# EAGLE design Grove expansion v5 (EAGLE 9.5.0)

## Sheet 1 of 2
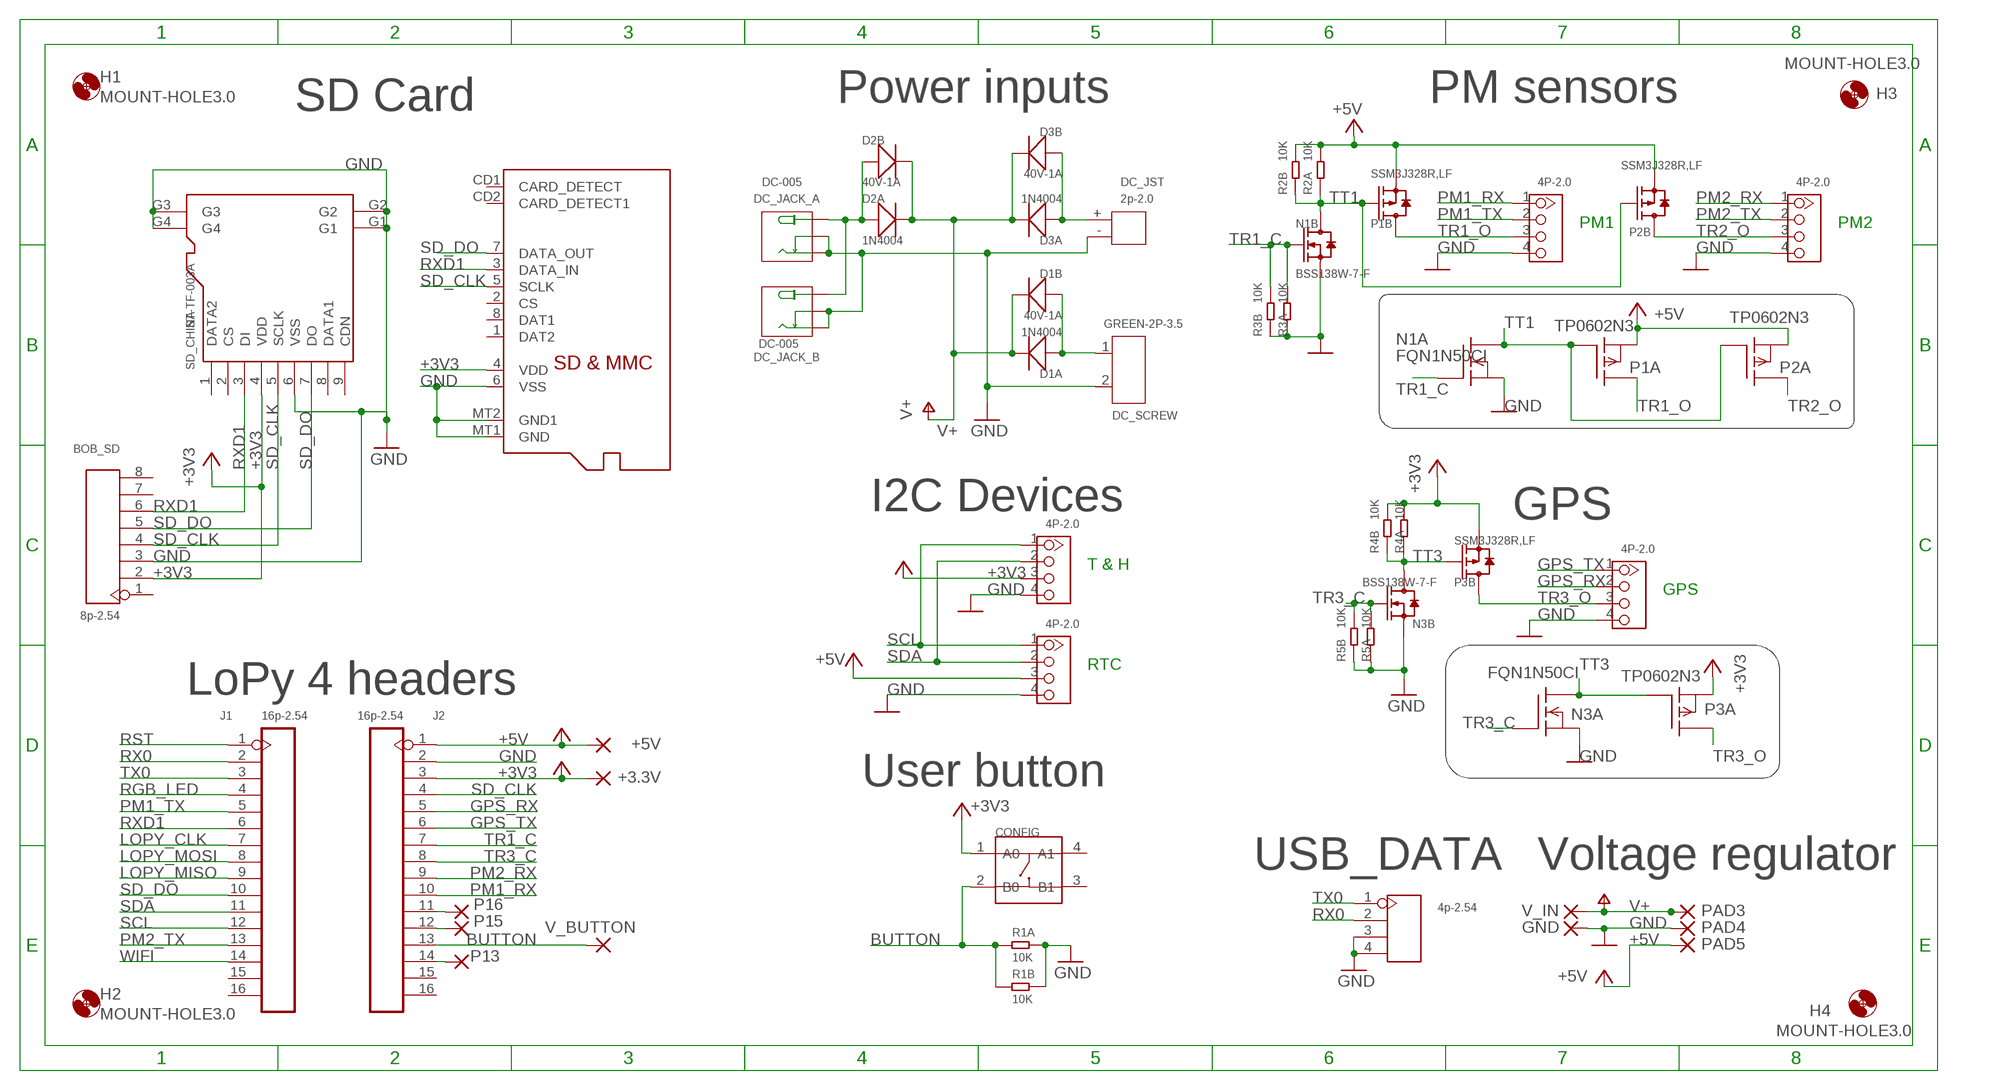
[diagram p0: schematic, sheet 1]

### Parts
+3.3V  3.3V  2,15/1,0  [2,15/1,0]
+5V  5V  2,15/1,0  [2,15/1,0]
BOB_SD  8p-2.54  DIP-BLACK-FEMALE-HEADER-VERT(8P-2.54)  [H8-2.54]
CONFIG  DIP-SWITCH-TACTILE-SPST-NO/TS-1109(4P-D6.0MM)'TS-1109'  [SW4-6.0X6.0X5.0MM]
D1A  1N4004  DIP-DIODE-400V-1A(DO-41)  [DO-41]
D1B  40V-1A  SMD-DIODE-SCHOTTKY-40V-1A(DO-214AC)  [DO-214AC]
D2A  1N4004  DIP-DIODE-400V-1A(DO-41)  [DO-41]
D2B  40V-1A  SMD-DIODE-SCHOTTKY-40V-1A(DO-214AC)  [DO-214AC]
D3A  1N4004  DIP-DIODE-400V-1A(DO-41)  [DO-41]
D3B  40V-1A  SMD-DIODE-SCHOTTKY-40V-1A(DO-214AC)  [DO-214AC]
DC_JACK_A  DC-005  CONN-POWER-JACK-2.1MM(DC-005)  [DCJ3P-14.2X11.0X9.0MM]
DC_JACK_B  DC-005  CONN-POWER-JACK-2.1MM(DC-005)  [DCJ3P-14.2X11.0X9.0MM]
DC_JST  2p-2.0  DIP-JST-2P-2.0  [H2-2.0-6X4.5MM]
DC_SCREW  GREEN-2P-3.5  SCREW-TERMINAL-GREEN(2P-3.5)  [H2-3.5-7.0X7.0MM]
GND  0V  2,15/1,0  [2,15/1,0]
GPS-(DIG)  4P-2.0  GROVE-CONNECTOR-DIP(4P-2.0)  [HW4-2.0]
H1  MOUNT-HOLE3.0  [3,0]
H2  MOUNT-HOLE3.0  [3,0]
H3  MOUNT-HOLE3.0  [3,0]
H4  MOUNT-HOLE3.0  [3,0]
J1  16p-2.54  DIP-BLACK-MALE-HEADER-VERT(16P-2.54)  [H16-2.54]
J2  16p-2.54  DIP-BLACK-MALE-HEADER-VERT(16P-2.54)  [H16-2.54]
N1A  FQN1N50CI  [TO92-INLINE]
N1B  BSS138W-7-F  SMD-MOSFET-N-CH-50V-200MA-BSS138W-7-F(SOT-23)  [SOT-23]
N3A  FQN1N50CI  [TO92-INLINE]
N3B  BSS138W-7-F  SMD-MOSFET-N-CH-50V-200MA-BSS138W-7-F(SOT-23)  [SOT-23]
P1A  TP0602N3  [TO-92]
P1B  SSM3J328R,LF  SMD-MOSFET-P-CH-20V-6A-SSM3J328R(SOT-23)  [SOT-23]
P2A  TP0602N3  [TO-92]
P2B  SSM3J328R,LF  SMD-MOSFET-P-CH-20V-6A-SSM3J328R(SOT-23)  [SOT-23]
P3A  TP0602N3  [TO-92]
P3B  SSM3J328R,LF  SMD-MOSFET-P-CH-20V-6A-SSM3J328R(SOT-23)  [SOT-23]
P13  2,15/1,0  [2,15/1,0]
P15  2,15/1,0  [2,15/1,0]
P16  2,15/1,0  [2,15/1,0]
PAD3  12V  1,6/0,8  [1,6/0,8]
PAD4  0V  1,6/0,8  [1,6/0,8]
PAD5  5V  1,6/0,8  [1,6/0,8]
PM1-(UART)  4P-2.0  GROVE-CONNECTOR-DIP(4P-2.0)  [HW4-2.0]
PM2-(UART)  4P-2.0  GROVE-CONNECTOR-DIP(4P-2.0)  [HW4-2.0]
R1A  10K  DIP-RES-10K-5%-1/4W(PR-D2.3XL6.5MM)  [PR-D2.3XL6.5MM]
R1B  10K  SMD-RES-10K-1%-1/10W(0603)  [R0603]
R2A  10K  DIP-RES-10K-5%-1/4W(PR-D2.3XL6.5MM)  [PR-D2.3XL6.5MM]
R2B  10K  SMD-RES-10K-1%-1/10W(0603)  [R0603]
R3A  10K  DIP-RES-10K-5%-1/4W(PR-D2.3XL6.5MM)  [PR-D2.3XL6.5MM]
R3B  10K  SMD-RES-10K-1%-1/10W(0603)  [R0603]
R4A  10K  DIP-RES-10K-5%-1/4W(PR-D2.3XL6.5MM)  [PR-D2.3XL6.5MM]
R4B  10K  SMD-RES-10K-1%-1/10W(0603)  [R0603]
R5A  10K  DIP-RES-10K-5%-1/4W(PR-D2.3XL6.5MM)  [PR-D2.3XL6.5MM]
R5B  10K  SMD-RES-10K-1%-1/10W(0603)  [R0603]
RTC-(I2C)  4P-2.0  GROVE-CONNECTOR-DIP(4P-2.0)  [HW4-2.0]
SD_CHINA  ST-TF-003A  MICRO-SD-CARD-SOCKET-9P(ST-TF-003A)  [MICRO-SD9+4P-SMD-16.1X14.5X1.85MM]
SD_UK  MICROSD  [MICROSD]
TH-(I2C)  4P-2.0  GROVE-CONNECTOR-DIP(4P-2.0)  [HW4-2.0]
USB_DATA  4p-2.54  DIP-BLACK-FEMALE-HEADER-VERT(4P-2.54)  [H4-2.54]
V_BUTTON  3.3V  2,15/1,0  [2,15/1,0]
V_IN  12V  2,15/1,0  [2,15/1,0]

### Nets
+3V3: +3.3V.1(P) BOB_SD.2 CONFIG.1(A0) J2.3 P3A.1(S) P3B.2(S) R4A.2 R4B.2 SD_CHINA.4(VDD) SD_UK.4(VDD) TH-(I2C).3
+5V: +5V.1(P) J2.1 P1A.1(S) P1B.2(S) P2A.1(S) P2B.2(S) PAD5.1(P) R2A.2 R2B.2 RTC-(I2C).3
BUTTON: CONFIG.2(B0) J2.13 R1A.1 R1B.1 V_BUTTON.1(P)
GND: BOB_SD.3 DC_JACK_A.-1(-) DC_JACK_A.-2(CDN) DC_JACK_B.-1(-) DC_JACK_B.-2(CDN) DC_JST.- DC_SCREW.2 GND.1(P) GPS-(DIG).4 J2.2 N1A.3(S) N1B.2(S) N3A.3(S) N3B.2(S) PAD4.1(P) PM1-(UART).4 PM2-(UART).4 R1A.2 R1B.2 R3A.1 R3B.1 R5A.1 R5B.1 RTC-(I2C).4 SD_CHINA.6(VSS) SD_CHINA.G1 SD_CHINA.G2 SD_CHINA.G3 SD_CHINA.G4 SD_UK.6(VSS) SD_UK.MT1(GND) SD_UK.MT2(GND1) TH-(I2C).4 USB_DATA.3 USB_DATA.4
GPS_RX: GPS-(DIG).2 J2.5
GPS_TX: GPS-(DIG).1 J2.6
JACK_V+: D2A.1(+) D2B.1(+) DC_JACK_A.+ DC_JACK_B.+
JST_V+: D3A.1(+) D3B.1(+) DC_JST.+
LOPY_CLK: J1.7
LOPY_MISO: J1.9
LOPY_MOSI: J1.8
P13: J2.14 P13.1(P)
P15: J2.12 P15.1(P)
P16: J2.11 P16.1(P)
PM1_RX: J2.10 PM1-(UART).1
PM1_TX: J1.5 PM1-(UART).2
PM2_RX: J2.9 PM2-(UART).1
PM2_TX: J1.13 PM2-(UART).2
RGB_LED: J1.4
RST: J1.1
RX0: J1.2 USB_DATA.2
RXD1: BOB_SD.6 J1.6 SD_CHINA.3(DI) SD_UK.3(DATA_IN)
SCL: J1.12 RTC-(I2C).1 TH-(I2C).1
SCREW_V+: D1A.1(+) D1B.1(+) DC_SCREW.1
SD_CLK: BOB_SD.4 J2.4 SD_CHINA.5(SCLK) SD_UK.5(SCLK)
SD_DO: BOB_SD.5 J1.10 SD_CHINA.7(DO) SD_UK.7(DATA_OUT)
SDA: J1.11 RTC-(I2C).2 TH-(I2C).2
TR1_C: J2.7 N1A.2(G) N1B.1(G) R3A.2 R3B.2
TR1_O: P1A.3(D) P1B.3(D) PM1-(UART).3
TR2_O: P2A.3(D) P2B.3(D) PM2-(UART).3
TR3_C: J2.8 N3A.2(G) N3B.1(G) R5A.2 R5B.2
TR3_O: GPS-(DIG).3 P3A.3(D) P3B.3(D)
TT1: N1A.1(D) N1B.3(D) P1A.2(G) P1B.1(G) P2A.2(G) P2B.1(G) R2A.1 R2B.1
TT3: N3A.1(D) N3B.3(D) P3A.2(G) P3B.1(G) R4A.1 R4B.1
TX0: J1.3 USB_DATA.1
V+: D1A.2(-) D1B.2(-) D2A.2(-) D2B.2(-) D3A.2(-) D3B.2(-) PAD3.1(P) V_IN.1(P)
WIFI: J1.14
Unconnected: BOB_SD.1 BOB_SD.7 BOB_SD.8 CONFIG.3(B1) CONFIG.4(A1) J1.15 J1.16 J2.15 J2.16 SD_CHINA.1(DATA2) SD_CHINA.2(CS) SD_CHINA.8(DATA1) SD_CHINA.9(CDN) SD_UK.1(DAT2) SD_UK.2(CS) SD_UK.8(DAT1) SD_UK.CD1(CARD_DETECT) SD_UK.CD2(CARD_DETECT1)

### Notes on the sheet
- SD Card | Power inputs | PM sensors
- PM1 | PM2
- I2C Devices | GPS
- T & H
- GPS
- RTC
- LoPy 4 headers
- User button
- Voltage regulator

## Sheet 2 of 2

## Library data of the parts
+3.3V +5V GND P13 P15 P16 V_BUTTON V_IN = wirepad:2,15/1,0: THROUGH-HOLE PAD
BOB_SD = OPL_Connector:DIP-BLACK-FEMALE-HEADER-VERT(8P-2.54): 320030061; MPN: F185-1108A1BSYC1
CONFIG = OPL_Switch:DIP-SWITCH-TACTILE-SPST-NO/TS-1109(4P-D6.0MM): 311020024
D1A D2A D3A = OPL_Discrete_Semiconductor:DIP-DIODE-400V-1A(DO-41): 304010008; MPN: 1N4004
D1B D2B D3B = OPL_Discrete_Semiconductor:SMD-DIODE-SCHOTTKY-40V-1A(DO-214AC): 304020027; MPN: 1N5819
DC_JACK_A DC_JACK_B = OPL_Connector:CONN-POWER-JACK-2.1MM(DC-005): 320120003; MPN: DC-005
DC_JST = OPL_Connector:DIP-JST-2P-2.0: 320110049
DC_SCREW = OPL_Connector:SCREW-TERMINAL-GREEN(2P-3.5): 320110028
GPS-(DIG) PM1-(UART) PM2-(UART) RTC-(I2C) TH-(I2C) = OPL_Connector:GROVE-CONNECTOR-DIP(4P-2.0): 320110033
H1-H4 = holes:MOUNT-HOLE: MOUNTING HOLE with drill center marker
J1 J2 = OPL_Connector:DIP-BLACK-MALE-HEADER-VERT(16P-2.54): 320020034; MPN: P125-1116A0BS116AX
N1A N3A = adafruit:FQN1N50C: N-Channel Enhancement MOSFET 500V, 0.4A, 6.0 Ohm
N1B N3B = OPL_Discrete_Semiconductor:SMD-MOSFET-N-CH-50V-200MA-BSS138W-7-F(SOT-23): 305030000; MPN: BSS138W-7-F
P1A P2A P3A = transistor-fet:TP0602N3: P-Channel Enhancement MOSFET -20V; -2A; 2,0Ohm
P1B P2B P3B = OPL_Discrete_Semiconductor:SMD-MOSFET-P-CH-20V-6A-SSM3J328R(SOT-23): 305030075; MPN: SSM3J328R,LF
PAD3-PAD5 = wirepad:1,6/0,8: THROUGH-HOLE PAD
R1A R2A R3A R4A R5A = OPL_Resistor:DIP-RES-10K-5%-1/4W(PR-D2.3XL6.5MM): 301020001; MPN: FHCFR-1/4W-103J
R1B R2B R3B R4B R5B = OPL_Resistor:SMD-RES-10K-1%-1/10W(0603): 301011970; MPN: RC0603FR-0710KL
SD_CHINA = OPL_Connector:MICRO-SD-CARD-SOCKET-9P(ST-TF-003A): 320090000; MPN: ST-TF-003A
SD_UK = adafruit:MICROSD: Micro-SD / Transflash card holder with SPI pinout For the 3M # 2908-05WB-MG and/or 4UCON #19656 push-push type
USB_DATA = OPL_Connector:DIP-BLACK-FEMALE-HEADER-VERT(4P-2.54): 320030017; MPN: F185-1104A1BSYA1

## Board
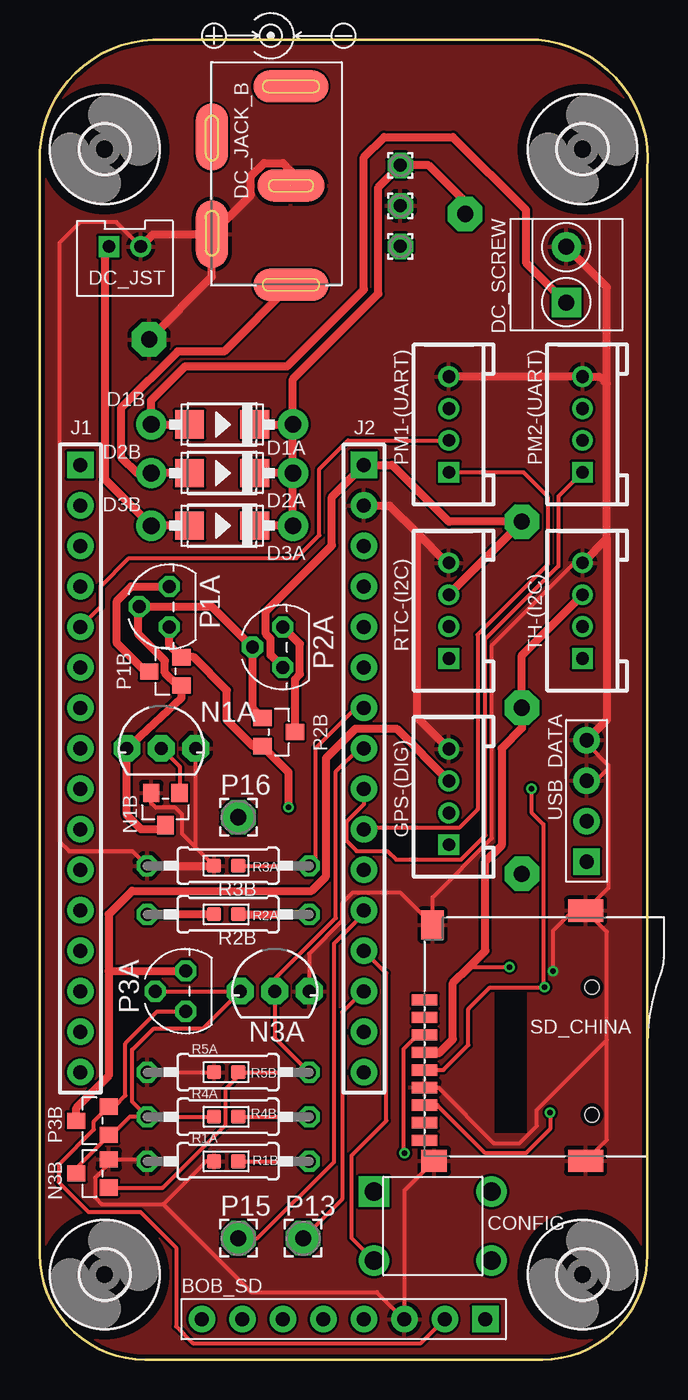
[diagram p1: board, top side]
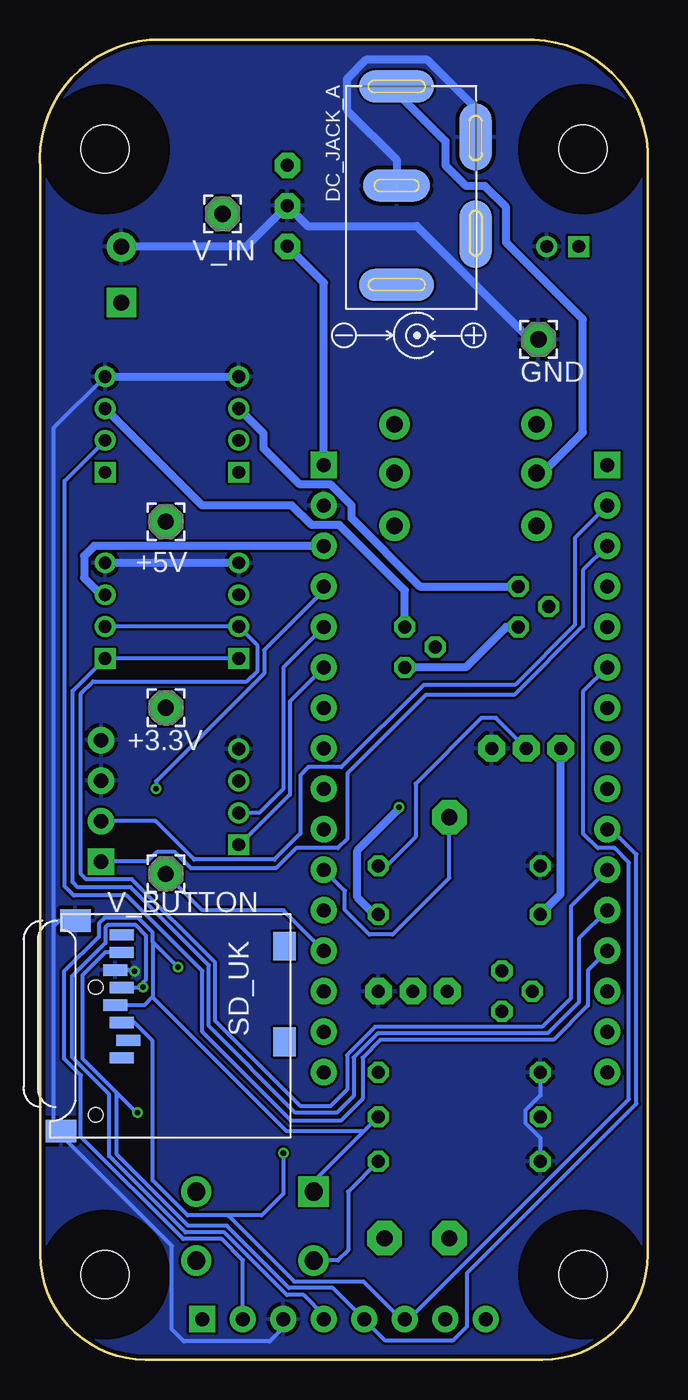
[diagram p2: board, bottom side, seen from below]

Size 38.13 x 82.8 mm. Coordinates in mm from the lower left corner, seen from the top.
Outline: 0,6.6 0,75.18 arc-90 7.11,82.8 31.24,82.8 arc-90 38.1,74.68 38.1,6.6 arc-90 31.5,0 6.6,0 arc-90 0,6.6
Copper layers (1*16): Top 0.035mm / dielectric 1.5mm / Bottom 0.035mm
Design rules "SeeedStudio_2layer_DRU_no_angle_20140221": minimum track width 6mil, minimum drill 12mil, track to track 6mil, track to pad 6mil, pad to pad 6mil, via to via 6mil, smd to smd 0mil, copper to edge 10mil, drill to drill 10mil, minimum pad ring 10mil, minimum via ring 6mil, stop-mask expansion 2mil, vias tented up to drill 100mil, thermal gap 10mil

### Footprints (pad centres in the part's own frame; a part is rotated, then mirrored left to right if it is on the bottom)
2,15/1,0 = drill 1.016 pad 2.159 octagon: 1 0,0
H8-2.54 = drill 0.889 pad 1.651 square: 1 0,8.89 | drill 0.889 pad 1.651: 2 0,6.35; 3 0,3.81; 4 0,1.27; 5 0,-1.27; 6 0,-3.81; 7 0,-6.35; 8 0,-8.89
SW4-6.0X6.0X5.0MM = drill 1.143 pad 1.905 square: 1 -3.683,2.159 | drill 1.143 pad 1.905: 2 -3.683,-2.159; 3 3.683,-2.159; 4 3.683,2.159
DO-41 = drill 1.041 pad 1.905: 1 -4.445,0; 2 4.445,0
DO-214AC = smd 1.8 x 1.77: 1 -2.042,0; 2 2.042,0
DCJ3P-14.2X11.0X9.0MM = smd 2 x 4.7: + 3.175,0 | smd 2 x 4.7 bottom: +1 3.175,0 | smd 2 x 4.2: -1 -3.048,0 | smd 4.2 x 2: -2 0,-4.953 | smd 2 x 4.2 bottom: -3 -3.048,0 | smd 4.2 x 2 bottom: -4 0,-4.953
H2-2.0-6X4.5MM = drill 0.8 pad 1.3 square: + -1,0.75 | drill 0.8 pad 1.3: - 1,0.75
H2-3.5-7.0X7.0MM = drill 1 pad 1.85 square: 1 -1.75,0 | drill 1 pad 1.85: 2 1.75,0
HW4-2.0 = drill 0.8 pad 1.27 square: 1 -3,0 | drill 0.8 pad 1.27: 2 -1,0; 3 1,0; 4 3,0
3,0 = hole 3: 0,0
H16-2.54 = drill 0.889 pad 1.651 square: 1 0,-19.05 | drill 0.889 pad 1.651: 2 0,-16.51; 3 0,-13.97; 4 0,-11.43; 5 0,-8.89; 6 0,-6.35; 7 0,-3.81; 8 0,-1.27; 9 0,1.27; 10 0,3.81; 11 0,6.35; 12 0,8.89; 13 0,11.43; 14 0,13.97; 15 0,16.51; 16 0,19.05
TO92-INLINE = drill 0.813 pad 1.676 octagon: 1 -2.159,0; 2 0,0; 3 2.159,0
SOT-23 = smd 1.016 x 1.143: 1 -0.889,-1.016; 2 0.889,-1.016; 3 0,1.016
TO-92 = drill 0.813 octagon: 1 -1.27,0; 2 0,1.905; 3 1.27,0
1,6/0,8 = drill 0.813 pad 1.6 octagon: 1 0,0
PR-D2.3XL6.5MM = drill 0.813 octagon: 1 -4.953,0; 2 5.207,0
R0603 = smd 0.889 x 0.889: 1 0,0.762; 2 0,-0.762
MICRO-SD9+4P-SMD-16.1X14.5X1.85MM = smd 1.6 x 0.7: 1 0,2.25; 2 0,1.15; 3 0,0.05; 4 0,-1.05; 5 0,-2.15; 6 0,-3.25; 7 0,-4.35; 8 0,-5.45; 9 0,-6.55 | smd 1.6 x 1.4: G1 0.6,-7.85 | smd 2.2 x 1.4: G2 10.1,-7.85; G3 10.1,7.85 | smd 1.4 x 1.8: G4 0.5,6.95 | hole 0.9: 10.5,-4.95; 10.5,3.05
MICROSD = smd 0.7 x 1.5: 1 9,-10.64; 2 7.9,-10.24; 3 6.8,-10.64; 4 5.7,-11.04; 5 4.6,-10.64; 6 3.5,-11.04; 7 2.4,-10.64; 8 1.3,-10.64 | smd 1.8 x 1.4: CD1 2,-0.44; CD2 8,-0.44 | smd 1.4 x 1.9: MT1 0.4,-13.54; MT2 13.6,-14.44
H4-2.54 = drill 0.889 pad 1.651 square: 1 0,3.81 | drill 0.889 pad 1.651: 2 0,1.27; 3 0,-1.27; 4 0,-3.81

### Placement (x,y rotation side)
+3.3V  30.23,40.89 0 bottom
+5V  30.23,52.58 0 bottom
BOB_SD  19.05,2.54 270 top
CONFIG  24.64,8.38 0 top
D1A  11.43,58.67 0 top
D1B  11.43,58.67 0 top
D2A  11.43,55.63 0 top
D2B  11.43,55.63 0 top
D3A  11.43,52.32 0 top
D3B  11.43,52.32 0 top
DC_JACK_A  15.75,76.71 90 bottom
DC_JACK_B  15.75,70.61 270 top
DC_JST  5.33,69.09 0 top
DC_SCREW  33.02,68.07 90 top
GND  6.86,64.01 0 bottom
GPS-(DIG)  25.65,35.31 90 top
H1  34.04,5.33 0 top
H2  4.06,75.95 0 top
H3  34.04,75.95 0 top
H4  4.06,5.33 0 top
J1  2.54,37.08 180 top
J2  20.32,37.08 180 top
N1A  7.62,38.35 0 top
N1B  7.87,34.54 180 top
N3A  14.73,23.11 0 top
N3B  3.3,11.68 90 top
P1A  8.13,47.24 90 top
P1B  7.87,43.18 90 top
P2A  15.24,44.7 90 top
P2B  14.99,39.37 270 top
P3A  9.14,23.11 90 top
P3B  3.3,14.99 90 top
P13  16.51,7.62 0 top
P15  12.45,7.62 0 top
P16  12.45,34.04 0 top
PAD3  22.61,74.93 90 top
PAD4  22.61,72.39 90 top
PAD5  22.61,69.85 90 top
PM1-(UART)  25.65,58.67 90 top
PM2-(UART)  34.04,58.67 90 top
R1A  11.94,12.45 180 top
R1B  11.68,12.45 270 top
R2A  11.68,27.94 0 top
R2B  11.68,27.94 90 top
R3A  11.68,30.99 0 top
R3B  11.68,30.99 90 top
R4A  11.68,15.24 0 top
R4B  11.68,15.24 90 top
R5A  11.68,18.03 0 top
R5B  11.68,18.03 90 top
RTC-(I2C)  25.65,46.99 90 top
SD_CHINA  24.13,20.32 0 top
SD_UK  22.35,27.94 270 bottom
TH-(I2C)  34.04,46.99 90 top
USB_DATA  34.29,35.05 180 top
V_BUTTON  30.23,30.48 0 bottom
V_IN  26.67,71.88 0 bottom

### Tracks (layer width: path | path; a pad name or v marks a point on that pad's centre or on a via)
+3V3  (via drill 0.35)
  Top 0.254: BOB_SD.2 23.89,1.03 9.6,1.03 8.55,2.08 8.55,7.03 6.31,9.27 3.04,9.27 1.18,11.13 1.18,12.23 3.39,14.44 3.39,14.95 P3B.2 4.66,15.88 5.36,16.58 5.36,19.84 7.37,21.84 P3A.1 | R4B.2 R4A.2 | 25.05,19.23 24.17,19.23 SD_CHINA.4 | 26.92,24.64 v29.46,24.64
  Top 0.508: 25.05,19.23 25.91,20.1 25.91,23.62 26.92,24.64 27.94,25.65 27.94,31.24 28.96,32.26 28.96,38.35 30.23,39.62 +3.3V.1 30.23,44.18 TH-(I2C).3
  Bottom 0.254: 31.05,26.22 31.05,22.77 31.07,22.75 | 31.07,22.75 31.58,22.24 SD_UK.4 | BOB_SD.2 25.4,6.25 26.73,7.58 29.15,7.58 35.56,13.99 35.56,17.85 36.61,18.9 36.61,24.35 34.43,26.53 34.43,27.36 34.07,27.72 31.97,27.72 31.05,26.8 31.05,26.22 | 31.07,22.75 22.65,14.33 17.83,14.33 16.91,15.24 R4A.2 20.95,11.18 CONFIG.1 | v29.46,24.64 31.05,26.22
  Bottom 0.508: TH-(I2C).3 34.3,47.99 35.35,49.04 35.35,50.43 34.73,51.05 J2.3
+5V  (via drill 0.35)
  Top 0.508: R2B.2 R2A.2 | RTC-(I2C).3 30.23,52.56 +5V.1 25.65,52.58 22.1,56.13 J2.1 18.31,54.13 18.31,51.08 14.17,46.94 14.17,45.53 14.48,45.23 14.48,44.2 P2A.1 | v15.61,34.66 15.61,36.84 P2B.2 13.39,38.48 11.73,40.13 11.73,41.99 9.65,44.07 P1B.2 8.13,44.83 P1A.1
  Bottom 0.508: J2.1 20.32,67.56 PAD5.1 | v15.61,34.66 15.61,34.54 18.21,31.94 18.21,29.01 17.14,27.94 R2A.2 | P1A.1 8.89,45.97 11.43,43.43 P2A.1
BUTTON
  Top 0.254: J2.13 21.73,24.24 21.73,14.99 19.56,12.81 19.56,7.62 CONFIG.2 | R1B.1 R1A.1
  Bottom 0.254: V_BUTTON.1 27.94,28.19 22.86,28.19 J2.13 | R1A.1 18.8,10.54 18.8,6.86 19.43,6.22 CONFIG.2
GND  (via drill 0.35)  (1 unrouted)
  Top 0.254: 24.73,12.82 SD_CHINA.G1 22.86,10.6 BOB_SD.3 22.86,2.5 21.13,4.23 13.26,4.23 7.74,9.75 | DC_JST.- 4.8,71.37 2.54,71.37 1.22,70.05 1.22,32.52 1.83,31.92 5.8,31.92 R3A.1 | USB_DATA.4 34.29,38.65 35.65,37.29 35.65,37.08 | 35.65,37.08 35.65,29.59 SD_CHINA.G3 | 11.23,18.03 R5B.1 R5A.1 | SD_CHINA.G3 35.56,26.84 35.56,20.07 | SD_CHINA.G3 33.44,28.17 32.19,26.92 v32.19,24.38 | SD_CHINA.G2 35.56,13.8 35.56,20.07 | SD_CHINA.6 24.99,17.07 28.48,13.58 30.07,13.58 31.16,14.67 31.16,15.67 35.56,20.07 | R1A.2 6.6,12.57 N3B.2 4.45,12.45 4.45,12.4 3.47,11.42 3.47,10.17 3.88,9.75 7.74,9.75 | TH-(I2C).4 33.53,49.99 28.35,44.81 28.35,32.72 24.63,29 SD_CHINA.G4 22.6,29.3 19.61,29.3 18.97,28.66 18.97,27.54 16.89,25.46 N3A.3 | R1B.2 10.43,12.45 7.74,9.75 | USB_DATA.3 34.89,36.32 35.65,37.08 | 6.73,35.31 N1B.2 6.99,34.92 7.28,34.63 8.5,34.63 8.91,34.21 8.91,32.99 R3B.1 9.78,32.13 N1A.3
  Top 0.508: DC_JST.- 7.11,70.61 DC_JACK_B.-2 | DC_JACK_B.-2 13.24,73.06 13.24,74.24 14.06,75.07 15.25,75.07 15.75,74.57 DC_JACK_B.-1 | N1B.2 7.06,35.64 | R3A.1 R3B.1 | 35.56,51.51 TH-(I2C).4 | 35.56,51.51 35.56,40.13 USB_DATA.4 | J2.2 21.93,53.59 23.66,51.86 | RTC-(I2C).4 25.53,49.99 23.66,51.86 | DC_SCREW.2 35.56,67.28 35.56,61.21 | PM1-(UART).4 PM2-(UART).4 35.1,61.67 35.56,61.21 | GPS-(DIG).4 23.66,40.3 23.66,51.86 | GND.1 10.79,67.95 DC_JACK_B.-2 | 35.56,51.51 35.56,61.21
  Bottom 0.254: PM2-(UART).4 37.27,58.44 37.27,27.18 | 37.27,27.18 37.27,14.67 36.95,14.34 SD_UK.MT2 36.79,14.09 29.84,7.14 29.84,1.89 29.1,1.14 23.71,1.14 22.86,1.99 BOB_SD.3 | SD_UK.6 32.25,24.44 v32.19,24.38 | R5A.1 6.73,16.57 7.67,15.63 7.67,14.85 6.73,13.91 R1A.2 | SD_UK.MT1 36.91,27.54 37.27,27.18
  Bottom 0.508: DC_JACK_A.-2 10.79,78.52 13.81,81.54 17.68,81.54 18.88,80.35 18.88,78.4 15.75,75.27 DC_JACK_B.-1 | RTC-(I2C).4 TH-(I2C).4 | GND.1 7.37,64.01 14.48,71.12 21.34,71.12 PAD4.1 25.17,69.82 DC_SCREW.2 | PM1-(UART).4 PM2-(UART).4 33.32,61.67
  pour Top: -1.27,85.34 -1.27,-1.02 39.37,-1.02 39.37,85.34
  pour Bottom: -2.79,86.61 -2.79,-2.29 40.64,-2.29 40.64,86.61
GPS_RX
  Bottom 0.254: J2.5 22.86,43.43 22.86,35.81 24.37,34.31 GPS-(DIG).2
GPS_TX
  Bottom 0.254: J2.6 22.45,41.3 22.45,35.46 25.61,32.31 GPS-(DIG).1
JACK_V+
  Top 0.508: D2B.1 D2A.1 6.1,55.63 5.08,56.64 5.08,59.69 8.64,63.25 11.56,63.25 DC_JACK_B.+
  Bottom 0.508: DC_JACK_A.+ 15.75,79.5 12.7,76.45 12.7,74.93 11.4,73.63 10.21,73.63 8.88,72.3 8.88,70.09 4.06,65.28 4.06,58.17 6.6,55.63 D2A.1
JST_V+
  Top 0.508: D3B.1 D3A.1 4.06,55.24 4.06,69.57 DC_JST.+
P13
  Top 0.254: J2.14 20.28,23.11 18.96,21.79 18.96,10.07 P13.1
P15
  Top 0.254: P15.1 13.65,7.62 18.45,12.42 18.45,26.11 20.32,27.98 J2.12
P16
  Bottom 0.254: J2.11 19,29.41 19,28.21 17.46,26.67 16,26.67 12.45,30.23 P16.1
PM1_RX
  Top 0.254: PM1-(UART).1 30.32,55.67 31.84,54.16 31.84,49.87 27.45,45.48 27.45,34.53 26.3,33.37 20.42,33.37 J2.10
PM1_TX
  Top 0.254: J1.5 3.81,47.24 3.81,48.51 5.59,50.29 16.09,50.29 17.53,51.72 17.53,55.88 19.32,57.67 PM1-(UART).2
PM2_RX
  Top 0.254: J2.9 20.32,34.84 19.21,33.73 19.21,32.56 19.86,31.92 21.8,31.92 22.34,31.37 26.42,31.37 27.94,32.89 27.94,45.21 32.51,49.79 32.51,54.15 PM2-(UART).1
PM2_TX
  Bottom 0.254: PM2-(UART).2 36.58,55.13 36.58,29.7 35.99,29.12 32.68,29.12 27.94,24.38 27.94,20.57 22.35,14.99 19.27,14.99 17.89,16.36 17.89,18.94 16.76,20.07 5.91,20.07 3.76,22.22 3.76,24.44 J1.13
RX0
  Bottom 0.254: J1.2 4.57,51.56 4.57,46.09 8.32,42.34 14.05,42.34 19.21,37.17 21.29,37.17 21.79,36.66 21.79,33 23.43,31.37 28.46,31.37 30.86,33.78 USB_DATA.2
RXD1  (via drill 0.35)
  Top 0.254: SD_CHINA.3 24.09,20.41 23.72,20.41 22.8,19.48 22.8,13.02 v22.86,12.95
  Bottom 0.254: SD_UK.3 32.95,21.18 32.23,21.18 31.05,20 31.05,11.24 28.87,9.05 26.33,9.05 | 26.33,9.05 22.19,4.91 17.83,4.91 15.46,2.54 BOB_SD.6 14.99,2.54 1.18,16.35 1.18,31.19 2.08,32.09 3.14,32.09 4.06,33.02 4.06,41.91 J1.6 | v22.86,12.95 22.86,10.41 24.22,9.05 26.33,9.05
SCL
  Bottom 0.254: J1.12 4.32,26.42 4.32,22.42 6.27,20.47 16.93,20.47 18.45,18.95 18.45,16.56 19.52,15.49 22.1,15.49 27.53,20.93 27.53,24.74 32.42,29.63 35.74,29.63 36.07,29.96 36.07,41.96 TH-(I2C).1 RTC-(I2C).1
SCREW_V+
  Top 0.508: D1B.1 D1A.1 6.99,60.2 9.12,62.33 15.51,62.33 20.32,67.15 20.32,75.44 21.59,76.71 25.91,76.71 30.48,72.14 30.48,68.83 32.99,66.32 DC_SCREW.1
SD_CLK  (via drill 0.35)
  Top 0.254: 31.59,23.44 v31.66,23.37 | v30.83,35.81 30.83,34.34 31.59,33.58 31.59,23.44 | SD_CHINA.5 25.3,18.17 26.88,19.75 26.88,22 28.22,23.35 31.49,23.35 31.59,23.44
  Bottom 0.254: BOB_SD.4 20.32,2.79 21.59,4.06 22.64,4.06 26.56,7.98 28.98,7.98 33.78,12.79 33.78,16.64 36.12,18.98 36.12,24.04 34.02,26.13 34.02,27.11 33.86,27.27 32.13,27.27 31.45,26.6 31.45,23.87 31.98,23.34 SD_UK.5 32.96,23.37 v31.66,23.37 | J2.4 20.32,48.26 24.06,44.52 24.06,43.05 30.83,36.28 v30.83,35.81
SD_DO  (via drill 0.35)
  Top 0.254: v32,15.49 32,14.48 30.48,12.95 27.94,12.95 24.92,15.97 SD_CHINA.7
  Bottom 0.254: SD_UK.7 33.03,25.58 34,25.58 35.46,24.12 35.46,18.9 33.3,16.74 | 33.3,16.74 33.3,12.88 28.82,8.4 26.4,8.4 22.51,4.51 19.75,4.51 BOB_SD.5 17.78,2.5 16.5,1.22 12.19,1.22 11.34,2.07 11.34,5.42 0.71,16.05 0.71,31.7 2.29,33.27 J1.10 | 33.3,16.74 32.06,15.49 v32,15.49
SDA
  Bottom 0.254: J1.11 4.83,28.45 4.83,22.67 6.62,20.88 17.1,20.88 18.86,19.12 18.86,16.96 19.91,15.9 21.76,15.9 27.13,21.26 27.13,24.91 32.36,30.14 35.23,30.14 35.56,30.47 35.56,41.78 34.79,42.55 25.14,42.55 24.47,43.22 24.47,44.8 RTC-(I2C).2 TH-(I2C).2
TR1_C
  Top 0.254: J2.7 19.81,40.89 17.27,38.35 17.27,31.24 17.02,30.99 R3A.2 R3B.2 | N1A.2 8.76,37.21 N1B.1
  Bottom 0.254: R3A.2 16.38,30.99 14.57,32.8 14.57,36.12 10.43,40.26 9.53,40.26 N1A.2
TR1_O
  Top 0.508: P1B.3 6.6,43.18 4.83,44.96 4.83,47.61 5.73,48.51 P1A.3
  Bottom 0.508: PM1-(UART).3 24.09,58.11 24.09,57.17 21.82,54.9 19.89,54.9 18.58,53.6 18.58,52.79 14.31,48.51 P1A.3
TR2_O
  Top 0.508: P2A.3 16.31,44.91 16.31,42.99 16,42.69 P2B.3
  Bottom 0.508: PM2-(UART).3 27.96,53.59 22.32,53.59 21.08,52.36 19.34,52.36 15.24,48.26 P2A.3
TR3_C
  Top 0.254: J2.8 20.03,38.35 18.57,36.89 18.57,27.71 14.73,23.88 N3A.2 14.73,20.19 R5A.2 12.7,18.03 | R5B.2 12.7,18.03 | 12.7,18.03 11.65,16.98 11.65,14.74 7.7,10.79 N3B.1
TR3_O
  Top 0.508: GPS-(DIG).3 22.37,39.59 19.81,39.59 17.96,37.73 17.96,30.33 17.04,29.41 5.79,29.41 4.32,27.94 4.32,24.38 | P3B.3 2.29,15.78 4.32,17.82 4.32,24.38 | 4.32,24.38 P3A.3
TT1
  Top 0.254: 7.62,33.27 N1B.3
  Top 0.508: R2B.1 R2A.1 | P2B.1 13.34,40.89 P2A.2 10.79,47.24 P1A.2 6.17,47.19 6.17,45.52 7.84,43.86 7.84,43.09 8.64,42.29 P1B.1 8.89,41.53 N1A.1 5.46,34.16 6.35,33.27 7.62,33.27
  Bottom 0.508: R2A.1 5.46,29.21 N1A.1
TT3
  Top 0.254: R4A.1 R4B.1 | N3B.3 2.29,12.02 4.32,14.05 P3B.1 4.52,14.1 5.68,15.25 5.69,15.24 R4A.1 | R4A.1 5.79,16.18 5.79,19.44 7.1,20.75 10.21,20.75 N3A.1 P3A.2
TX0
  Bottom 0.254: USB_DATA.1 31.39,31.24 30.79,31.84 29.66,31.84 28.65,30.82 23.32,30.82 22.05,32.09 19.43,32.09 18.85,32.68 18.85,36.78 13.92,41.71 8.38,41.71 4.06,46.02 4.06,49.53 J1.3
V+
  Top 0.508: D1B.2 D1A.2 | D2A.2 D2B.2 | D3B.2 D3A.2 D2A.2 | D2A.2 D1A.2 | D1A.2 15.88,61.51 21.23,66.87 21.23,73.56 PAD3.1 24.38,74.93 26.67,72.64 V_IN.1

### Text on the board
silktop: PyonAir V5 | 6.5 - 40 V | . | + | + | - | V-reg | + | - | Wires in | + | LoPy / LED | +5V | +5V | + | +5V | 3V3 | S | S | - GND | S | GND | 3V3 | - RX - | TX | V_Button | S | S | x / x | x / x | DI | DO | CLK | GND | 3V3
silkbottom: + | + | - | CC-BY-SA | + | - | + | pyonair.org | University of / Southampton | https://github.com/pyonair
